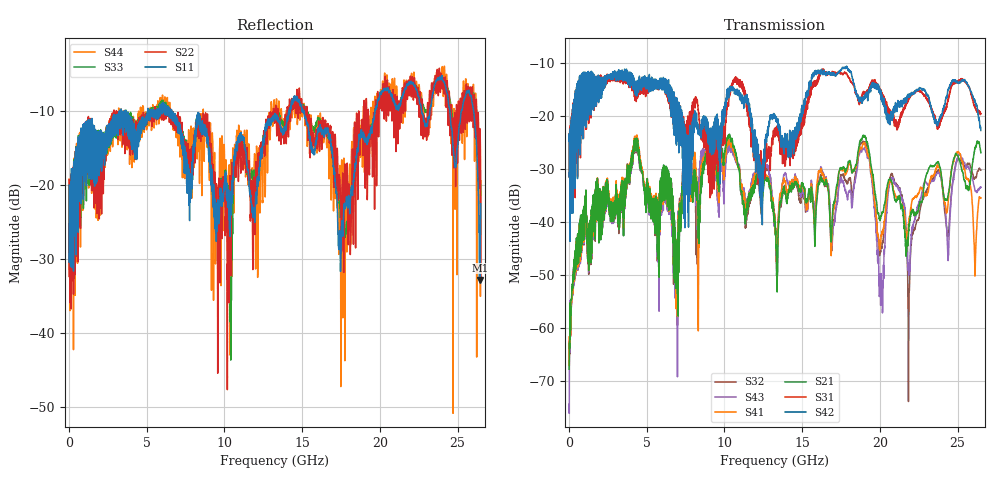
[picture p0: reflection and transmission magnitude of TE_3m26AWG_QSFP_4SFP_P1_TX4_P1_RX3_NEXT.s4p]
!Agilent Technologies,N5222A,MY51421691,A.10.00.00
!Agilent N5222A: A.10.00.00
!Date: Friday, January 30, 2015 12:34:41
!Correction: S11(Full 4 Port(1,2,3,4))
!S12(Full 4 Port(1,2,3,4))
!S13(Full 4 Port(1,2,3,4))
!S14(Full 4 Port(1,2,3,4))
!S21(Full 4 Port(1,2,3,4))
!S22(Full 4 Port(1,2,3,4))
!S23(Full 4 Port(1,2,3,4))
!S24(Full 4 Port(1,2,3,4))
!S31(Full 4 Port(1,2,3,4))
!S32(Full 4 Port(1,2,3,4))
!S33(Full 4 Port(1,2,3,4))
!S34(Full 4 Port(1,2,3,4))
!S41(Full 4 Port(1,2,3,4))
!S42(Full 4 Port(1,2,3,4))
!S43(Full 4 Port(1,2,3,4))
!S44(Full 4 Port(1,2,3,4))
!S4P File: Measurements: <S11,S12,S13,S14>,
!<S21,S22,S23,S24>,
!<S31,S32,S33,S34>,
!<S41,S42,S43,S44>:
# Hz S  dB  R 50.0
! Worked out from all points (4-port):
!   2650 points, 10 MHz to 26.5 GHz, reference 50 ohm
!   strongest paths, dB at 10 MHz, 6.63 GHz, 13.26 GHz, 19.88 GHz, 26.5 GHz:
!     S42: -24.9, -15.8, -19.9, -14.0, -22.8
!     S31: -24.8, -19.1, -23.3, -14.9, -19.7
!     S21: -67.9, -33.8, -40.1, -38.4, -27.0
!     S41: -61.8, -34.0, -39.3, -42.6, -35.6
!     S43: -74.5, -34.7, -40.3, -45.3, -33.5
!     S32: -65.5, -34.8, -39.9, -43.7, -30.3
!   lowest |S11| = -32.8 dB at 26.43 GHz (marker M1), VSWR 1.05, Z = 51.9 - j1.33 ohm
!   |S11| at or under -10 dB: start of sweep to 3.24 GHz; 6.606 GHz to 14.16 GHz (7.549 GHz wide, 72.7 % of centre); 15.11 GHz to 19.68 GHz (4.573 GHz wide, 26.3 % of centre)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
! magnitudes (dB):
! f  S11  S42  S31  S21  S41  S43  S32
! 10 MHz  -20.0  -24.9  -24.8  -67.9  -61.8  -74.5  -65.5
! 4.3 GHz  -12.7  -13.9  -14.8  -24.9  -24.5  -25.0  -25.3
! 6.89 GHz  -11.8  -19.9  -22.8  -46.0  -45.7  -45.2  -44.1
! 18.99 GHz  -13.9  -16.7  -15.7  -23.9  -25.3  -26.2  -25.1
! 21.85 GHz  -6.1  -16.5  -16.9  -41.6  -40.6  -49.5  -62.6
! 26.43 GHz  -32.8  -21.9  -19.4  -25.8  -35.6  -33.6  -30.0
! 26.5 GHz  -22.5  -22.8  -19.7  -27.0  -35.6  -33.5  -30.3
